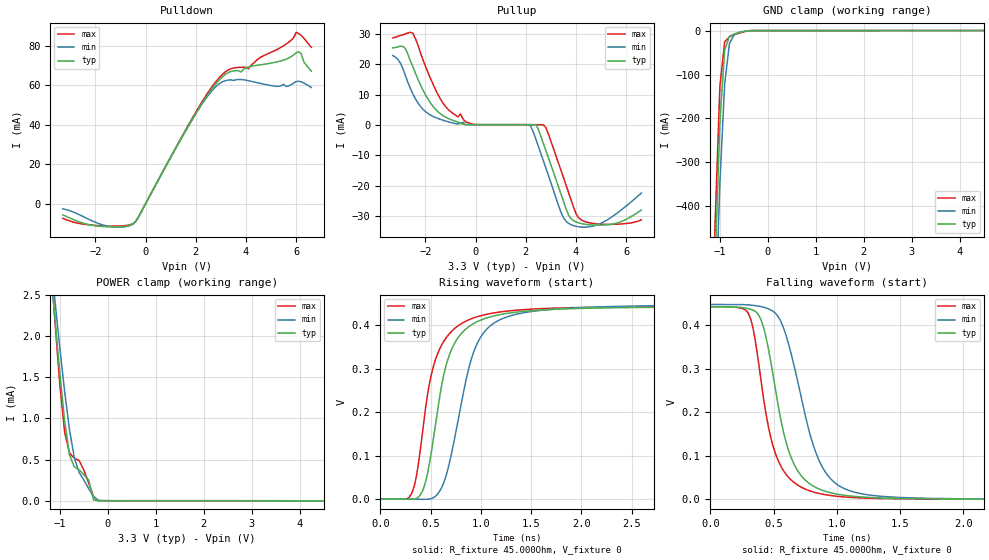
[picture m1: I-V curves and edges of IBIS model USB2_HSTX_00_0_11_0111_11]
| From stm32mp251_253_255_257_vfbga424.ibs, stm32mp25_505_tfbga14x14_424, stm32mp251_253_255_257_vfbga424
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[Model] USB2_HSTX_00_0_11_0111_11
Model_type   Output
Polarity   Non-Inverting
Enable   Active-High
C_comp   8.036pF   7.631pF   8.569pF
Vmeas = 200.000mV
Vref = 200.000mV
Rref = 45Ohms
Cref = 0pF
[Model Spec]
Vmeas   200.000mV   200.000mV   200.000mV
Vref   200.000mV   200.000mV   200.000mV
| This model is not intended for timing simulations.
| Warnings about Cref, Vref & Rref can be ignored
[Temperature Range]   25.000   125.000   -40.000
[Voltage Range]   3.300V   3.070V   3.630V
[GND Clamp Reference]   0.00V   0.00V   0.00V
[Pulldown Reference]   0.00V   0.00V   0.00V
[POWER Clamp Reference]   3.300V   3.070V   3.630V
[Pullup Reference]   3.300V   3.070V   3.630V
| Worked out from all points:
|   slope of the pulldown table from 0 to 0.495 V, typ, clamps not added: 42.6 ohm
|   GND clamp passes 1 mA (typ) near -0.43 V on its own axis
|   POWER clamp passes 1 mA (typ) near -0.91 V on its own axis
|   rising waveform, R_fixture 45.000Ohm, V_fixture 0: 20-80 % time 234ps typ, 270ps min, 225ps max; typ from 0 V to 0.442 V
|   falling waveform, R_fixture 45.000Ohm, V_fixture 0: 20-80 % time 196ps typ, 242ps min, 176ps max; typ from 0.442 V to 0 V
[GND Clamp]
-3.3V     -11.02A    -10.62A    -11.32A
-1.2V     -931.6mA   -1.049A    -855.7mA
-1.1V     -533.1mA   -671.7mA   -440.2mA
-1V       -209.4mA   -347mA     -127.3mA
-900mV    -44.44mA   -121.7mA   -25.6mA
-800mV    -13.15mA   -29.48mA   -14.15mA
-700mV    -7.742mA   -9.125mA   -9.769mA
-500mV    -2.127mA   -1.981mA   -2.894mA
-300mV    -19.45uA   -62.22uA   -13.64uA
6.6V      10.37uA    26.59uA    21.05uA
[Power Clamp]
-3.3V     3.206A     2.175A     4.855A
-1.2V     2.88mA     3.008mA    2.969mA
-1.1V     2.195mA    2.419mA    2.156mA
-1V       1.545mA    1.852mA    1.406mA
-900mV    967.9uA    1.324mA    831.4uA
-800mV    558.5uA    864.6uA    580.3uA
-700mV    412uA      525.9uA    517uA
-600mV    376.6uA    345uA      488.5uA
-400mV    254.2uA    146.6uA    216.8uA
-300mV    11.21uA    52.87uA    53.51uA
-100mV    94.8nA     984.9nA    361.1nA
6.6V      -2.795uA   -5.18uA    -3.59uA
[Pulldown]
-3.3V     -5.671mA   -2.581mA   -7.449mA
-1.6V     -11.64mA   -11.09mA   -11.31mA
-500mV    -10.25mA   -10.32mA   -10.1mA
1.9V      43.42mA    43.46mA    44.13mA
2.9V      62.15mA    60.37mA    63.26mA
3.4V      66.87mA    62.63mA    68.29mA
4.1V      69.19mA    62.19mA    68.26mA
4.5V      70.11mA    61.06mA    73.4mA
5.6V      73.12mA    59.29mA    80.76mA
6V        76.31mA    61.79mA    86.69mA
6.1V      76.87mA    61.93mA    85.99mA
6.6V      66.99mA    58.79mA    79.1mA
[Pullup]
-3.3V     25.41mA    22.87mA    28.68mA
-2.8V     25.23mA    16.38mA    30mA
-2.5V     19.29mA    10.28mA    30.27mA
-1.7V     6.185mA    2.829mA    13.54mA
-1.2V     2.602mA    1.31mA     6.112mA
-400mV    111.7uA    77.66uA    1.021mA
2.2V      68.63uA    -465.1uA   104.8uA
2.4V      56.24uA    -4.685mA   90.82uA
2.8V      -8.459mA   -14.22mA   -920uA
3.7V      -29.65mA   -32.41mA   -22.19mA
4.3V      -32.64mA   -33.68mA   -31.68mA
6.6V      -28.04mA   -22.46mA   -31.3mA
[Ramp]
R_load=45.000Ohm
dV/dt_r   633.020mV/1.005ns  601.226mV/1.010ns  686.730mV/960.000ps
dV/dt_f   635.187mV/225.000ps  604.107mV/285.000ps  688.533mV/210.000ps
[Rising waveform]
R_fixture=45.000Ohm
V_fixture=0
0s        452.2nV    3.129uV    468nV
320ps     -486.7uV   -405.8uV   17.36mV
370ps     3.022mV    -585.3uV   67.33mV
450ps     39.3mV     -570.4uV   209mV
590ps     234.5mV    18.02mV    345.2mV
760ps     367mV      164.1mV    396.6mV
920ps     403.1mV    332.8mV    416.5mV
1.09ns    419.4mV    398.1mV    427.1mV
2.36ns    440.8mV    443.8mV    442.2mV
9.9ns     442.5mV    448.1mV    442.6mV
[Falling waveform]
R_fixture=45.000Ohm
V_fixture=0
0s        441.9mV    447.5mV    442.1mV
310ps     437.2mV    446.4mV    421mV
420ps     395.5mV    441.2mV    232.7mV
530ps     226.1mV    422mV      93.26mV
680ps     70.53mV    284.7mV    34.71mV
810ps     30.96mV    127.5mV    17.2mV
930ps     16.6mV     54.11mV    9.62mV
1.16ns    6.185mV    14.88mV    3.624mV
1.71ns    1.151mV    2.415mV    840.6uV
9.9ns     14.44uV    30.35uV    5.266uV
